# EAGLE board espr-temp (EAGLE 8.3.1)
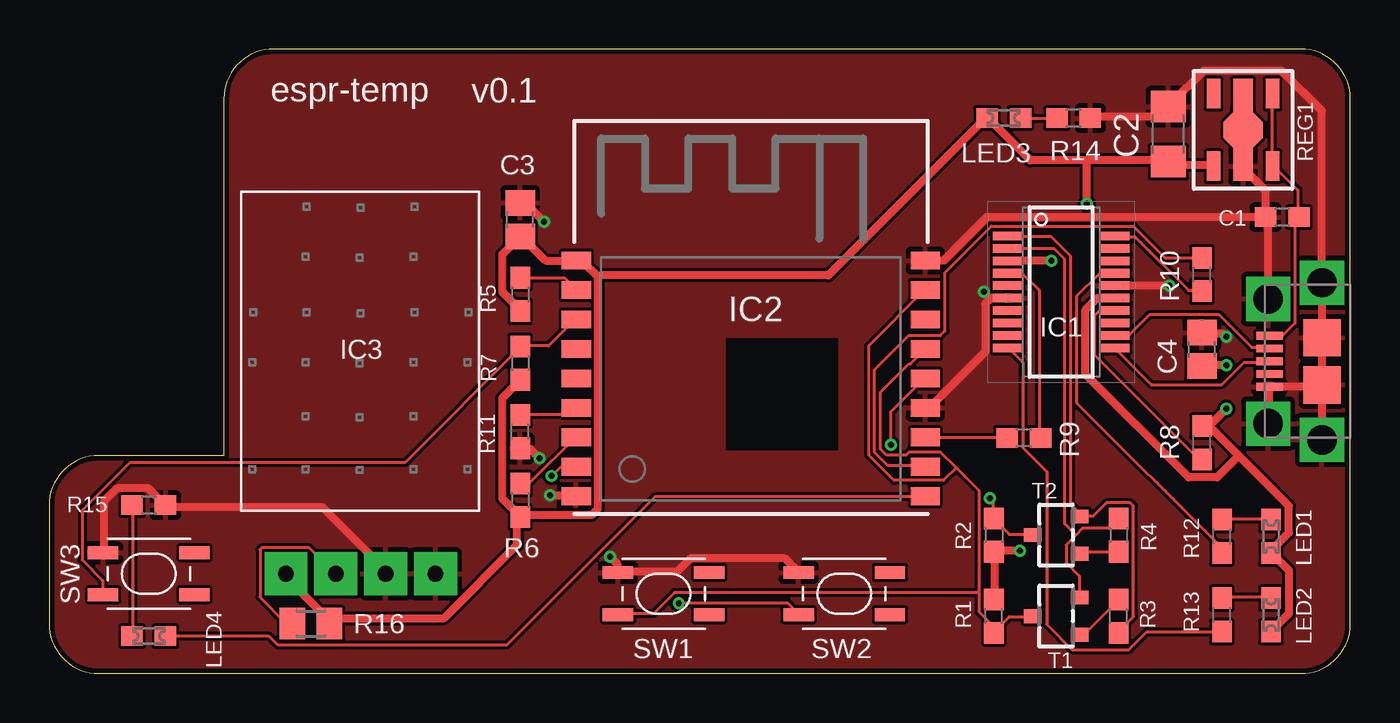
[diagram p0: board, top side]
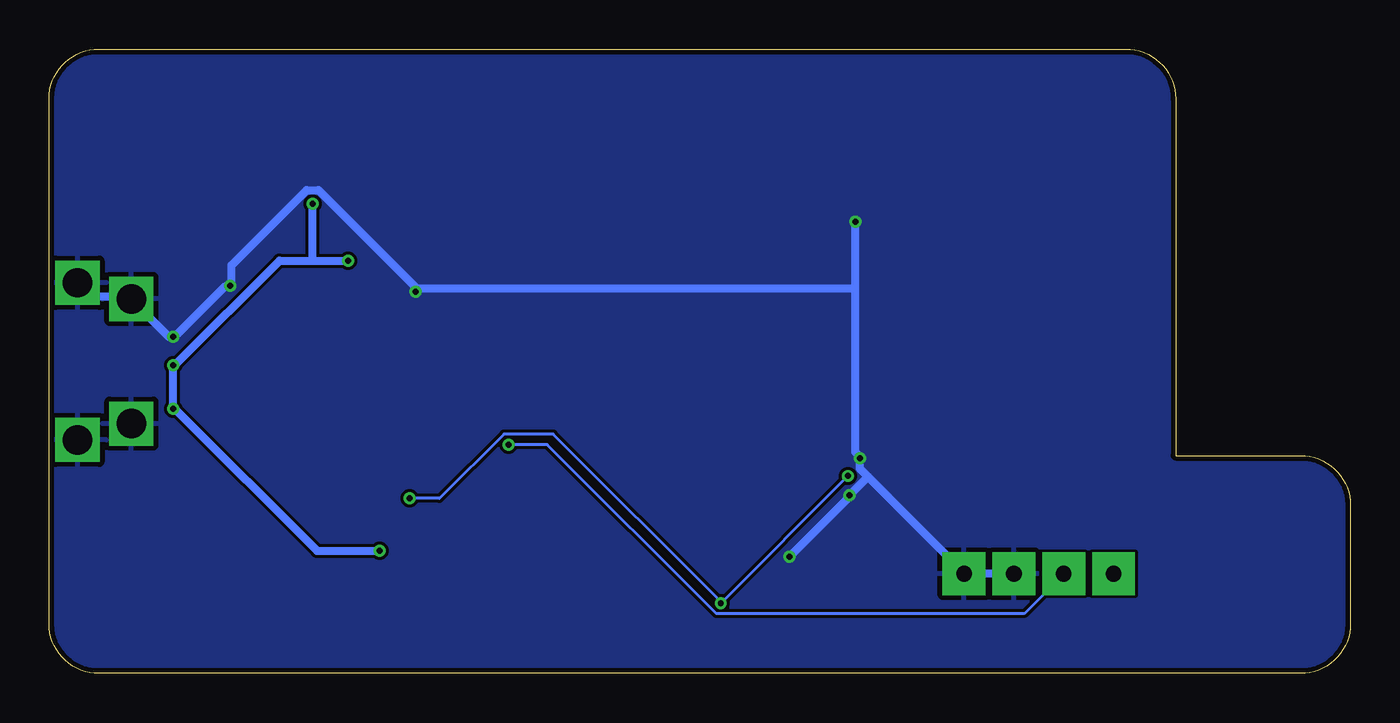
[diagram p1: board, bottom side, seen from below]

Size 66.3 x 31.8 mm. Coordinates in mm from the lower left corner, seen from the top.
Outline: 8.9,11.1 2.54,11.1 arc90 0,8.56 0,2.54 arc90 2.54,0 63.76,0 arc90 66.3,2.54 66.3,29.26 arc90 63.76,31.8 11.44,31.8 arc90 8.9,29.26 8.9,11.1
Copper layers (1*16): Top 0.035mm / dielectric 1.5mm / Bottom 0.035mm
Design rules "SeeedStudio_2layer_DRU_no_angle_20140221": minimum track width 6mil, minimum drill 12mil, track to track 6mil, track to pad 6mil, pad to pad 6mil, via to via 6mil, smd to smd 0mil, copper to edge 10mil, drill to drill 10mil, minimum pad ring 10mil, minimum via ring 6mil, stop-mask expansion 2mil, vias tented up to drill 100mil, thermal gap 10mil
Net classes: 1 GND: width 0.406 mm, drill 0.102 mm, clearance 0.127 mm; 2 3V3: width 0.406 mm, drill 0.102 mm, clearance 0.127 mm

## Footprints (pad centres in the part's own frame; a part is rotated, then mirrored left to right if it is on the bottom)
C1608 = smd 1.1 x 1: 1 -0.85,0; 2 0.85,0
C3216 = smd 1.6 x 1.8: 1 -1.4,0; 2 1.4,0
C2012 = smd 1.3 x 1.5: 1 -0.85,0; 2 0.85,0
SOP64P599X175-20N = smd 1.526 x 0.435: 1 -2.712,2.858; 2 -2.712,2.222; 3 -2.712,1.588; 4 -2.712,0.952; 5 -2.712,0.318; 6 -2.712,-0.318; 7 -2.712,-0.952; 8 -2.712,-1.588; 9 -2.712,-2.222; 10 -2.712,-2.858; 11 2.712,-2.858; 12 2.712,-2.222; 13 2.712,-1.588; 14 2.712,-0.952; 15 2.712,-0.318; 16 2.712,0.318; 17 2.712,0.952; 18 2.712,1.588; 19 2.712,2.222; 20 2.712,2.858
FRONT-FACE = smd 1.485 x 0.9: 1 -8.893,4.9; 2 -8.893,3.4; 3 -8.893,1.9; 4 -8.893,0.4; 5 -8.893,-1.1; 6 -8.893,-2.6; 7 -8.893,-4.1; 8 -8.893,-5.6; 9 -8.893,-7.1; 10 8.893,-7.1; 11 8.893,-5.6; 12 8.893,-4.1; 13 8.893,-2.6; 14 8.893,-1.1; 15 8.893,0.4; 16 8.893,1.9; 17 8.893,3.4; 18 8.893,4.9
AM2320 = drill 0.8 pad 2.184 square: GND 1.27,-11.43; SCL 3.81,-11.43; SDA -1.27,-11.43; VDD -3.81,-11.43
C1608' = smd 1.1 x 1: A 0.85,0; C -0.85,0
R1608 = smd 1.1 x 1: 1 -0.85,0; 2 0.85,0
M0805 = smd 1.3 x 1.6: 1 -0.95,0; 2 0.95,0
SOT-89-5 = smd 0.7 x 1.5: 1 -1.5,-1.85; 3 1.5,-1.85; 4 1.5,1.85; 5 -1.5,1.85 | smd 1 x 1.5: 2 0,-1.85; 2_1 0,1.85 | smd 0.8 x 0.8: 2_0 0,0; 2_4 -0.6,0; 2_5 0.6,0 | smd 1 x 0.5: 2_2 0,0.9; 2_7 0,-0.9 | smd 1.41 x 1.41 rotated 45: 2_3 0,0.4; 2_6 0,-0.4
SKRPACE010 = smd 1.55 x 0.65: 1 -2.325,1.075; 2 2.325,1.075; 3 -2.325,-1.075; 4 2.325,-1.075
SOT346 = smd 0.7 x 0.9: 1 -0.95,-1.2; 2 0.95,-1.2; 3 0,1.2
ZX62B5PA = smd 0.4 x 1.35: D+ 0,4.125; D- 0.65,4.125; GND -1.3,4.125; ID -0.65,4.125; VBUS 1.3,4.125 | drill 1.499 pad 2.032 square: SLD1 -3.175,4.191; SLD2 3.175,4.191; SLD3 -4,1.45; SLD6 4,1.45 | smd 1.9 x 1.9: SLD4 -1.2,1.45; SLD5 1.2,1.45

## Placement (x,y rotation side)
C1  0.39u  [C1608]  62.83,23.24 180 top
C2  4.7u  [C3216]  57.02,27.47 90 top
C3  0.1u  [C2012]  24,23.11 90 top
C4  0.1u  [C2012]  58.74,16.51 90 top
IC1  FT231XS-R  [SOP64P599X175-20N]  51.56,19.43 0 top
IC2  ESP-WROOM-02  [FRONT-FACE]  35.75,16.13 0 top
IC3  AM2320  [AM2320]  15.88,16.51 0 top
LED1  [C1608']  62.26,6.99 270 top
LED2  [C1608']  62.26,2.98 270 top
LED3  [C1608']  48.64,28.3 180 top
LED4  [C1608']  5.08,1.91 0 top
R1  10k  [R1608]  48.13,2.92 90 top
R2  10k  [R1608]  48.13,7.05 270 top
R3  10k  [R1608]  54.48,2.92 90 top
R4  10k  [R1608]  54.48,7.05 270 top
R5  10k  [R1608]  24,19.3 270 top
R6  10k  [R1608]  24,8.83 270 top
R7  10k  [R1608]  24,15.81 270 top
R8  10k  [R1608]  58.74,11.75 90 top
R9  470  [R1608]  49.66,12 180 top
R10  470  [R1608]  58.74,20.32 90 top
R11  10k  [R1608]  24,12.32 90 top
R12  1k  [R1608]  59.75,6.99 90 top
R13  1k  [R1608]  59.75,2.98 90 top
R14  10k  [R1608]  52.2,28.28 180 top
R15  1k  [R1608]  5.08,8.57 180 top
R16  4.7k  [M0805]  13.34,2.54 180 top
REG1  NJM2884U1  [SOT-89-5]  60.83,27.69 180 top
SW1  [SKRPACE010]  31.31,4.06 0 top
SW2  [SKRPACE010]  40.51,4.06 0 top
SW3  [SKRPACE010]  5.08,5.08 0 top
T1  [SOT346]  51.31,2.92 90 top
T2  [SOT346]  51.31,7.05 90 top
USB1  MICRO-USB  [ZX62B5PA]  66.3,15.9 90 top

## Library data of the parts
C1-C4 R16 = rcl
IC1 = FT231XS-R; DESCRIPTION: FTDI Chip FT231XS-R, Interface RS232, RS422, RS485, SIE, UART 3MBd, 5 V, 20-pin, SSOP; HEIGHT: 1.7526mm; MANUFACTURER_NAME: FTDI Chip; MANUFACTURER_PART_NUMBER: FT231XS-R; RS_PART_NUMBER: 7570032P
IC2 = esp-wroom-02
IC3 = am2320
LED1-LED4 = led-smd
R1-R15 = registors
REG1 = regulator
SW1-SW3 = switches
T1 T2 = transistors
USB1 = usb-connector

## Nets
+3V3 [3V3]: C2.1 C3.1 C4.1 IC1.3 IC1.15 IC2.1 IC3.VDD LED1.A LED2.A LED3.A R1.2 R2.2 R5.2 R6.2 R7.2 R8.2 R16.1 REG1.4
CBUS1: IC1.17 R12.1
CBUS2: IC1.10 R13.1
D+: IC1.11 USB1.D+
D-: IC1.12 USB1.D-
DTR: IC1.1 R3.1 T2.2
GND [GND]: C1.2 C2.2 C3.2 C4.2 IC1.6 IC1.16 IC2.9 IC2.13 IC2.18 IC3.GND IC3.SCL R11.1 R14.1 R15.1 REG1.2_1 SW1.1 SW2.1 SW3.1 USB1.GND USB1.SLD1 USB1.SLD2 USB1.SLD3 USB1.SLD4 USB1.SLD5 USB1.SLD6
IO0: IC2.8 R2.1 SW2.3 T2.3
IO4: IC2.10 LED4.A
IO5: IC2.14 IC3.SDA R16.2
N$1: IC2.2 R5.1
N$2: LED4.C R15.2
N$3: IC2.7 R6.1
N$4: C1.1 REG1.1 REG1.5 USB1.VBUS
N$5: LED1.C R12.2
N$6: R3.2 T1.1
N$7: R4.2 T2.1
N$8: LED2.C R13.2
N$9: LED3.C R14.2
N$10: IC2.12 R9.2
N$11: IC2.11 R10.2
N$12: IC2.6 R11.2
N$14: IC1.14 R8.1
N$16: IC2.3 R7.1 SW3.3
RESET: IC2.15 IC2.17 R1.1 SW1.3 T1.3
RTS: IC1.2 R4.1 T1.2
RXD: IC1.4 R9.1
TXD: IC1.20 R10.1

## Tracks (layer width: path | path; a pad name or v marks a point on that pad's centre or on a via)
+3V3  (via drill 0.3)
  Top 0.406: R5.2 24,18.52 23.09,19.43 23.09,21.34 C3.1 24.16,22.17 25.3,21.03 26.82,21.03 IC2.1 27.05,20.95 27.2,20.95 27.96,20.19 | R6.2 24,8 23.09,8.91 23.09,14.02 24,14.94 R7.2 | IC3.VDD 12.12,5.03 12.12,4.88 14.25,2.74 14.25,2.59 R16.1 14.4,2.82 20.12,2.82 23.85,6.55 23.85,7.85 R6.2 | 27.96,20.19 27.96,8.38 27.66,8.08 24.16,8.08 R6.2 | 52.88,26.14 57,26.14 C2.1 57.15,25.91 59.28,25.91 REG1.4 | 52.88,26.14 49.99,26.14 47.85,28.27 LED3.A 47.62,28.19 39.7,20.27 28.12,20.27 27.96,20.19 | R1.2 48.16,3.81 48.16,6.17 R2.2 48.31,6.25 v49.45,6.25 | LED2.A 62.33,2.21 63.17,3.05 63.17,5.26 62.33,6.1 LED1.A 62.33,6.33 63.17,7.16 63.17,8.53 60.62,11.09 | 60.62,11.09 59.13,12.57 58.75,12.57 R8.2 59.21,12.72 v59.97,13.49 | v59.97,15.7 58.75,15.7 C4.1 | v51.05,21.03 48.92,21.03 IC1.3 | 60.62,11.09 59.51,9.98 58.06,9.98 52.81,15.24 52.81,18.52 53.42,19.13 54.25,19.13 IC1.15 | v52.88,23.93 52.88,26.14
  Bottom 0.406: 52.88,21.03 54.56,21.03 59.82,15.77 v59.97,15.7 v59.97,13.49 59.82,13.41 52.65,6.25 v49.45,6.25 | 52.88,21.03 v51.05,21.03 | 52.88,21.03 v52.88,23.93
CBUS1
  Top 0.152: R12.1 59.74,6.17 59.74,6.4 52.35,13.79 52.35,19.2 53.49,20.34 54.25,20.34 IC1.17
CBUS2
  Top 0.152: R13.1 55.93,2.13 55.02,1.22 52.12,1.22 50.83,2.52 50.83,10.29 49.61,11.51 49.61,15.85 48.92,16.54 IC1.10
D+
  Top 0.152: USB1.D+ 62.1,15.85 60.88,15.85 59.74,14.71 56.16,14.71 54.33,16.54 IC1.11
D-
  Top 0.152: USB1.D- 62.1,16.61 61.27,16.61 59.59,18.29 56.08,18.29 55.02,17.22 54.33,17.22 IC1.12
DTR
  Top 0.152: R3.1 54.48,2.13 55.24,2.9 55.24,8.53 55.09,8.69 53.87,8.69 53.19,8 52.58,8 T2.2 52.58,8.08 52.05,8.61 52.05,21.26 51.05,22.25 48.92,22.25 IC1.1
GND  (via drill 0.3)
  Top 0.406: C1.2 61.95,23.24 61.95,24.61 60.88,25.68 60.88,25.83 REG1.2_1 | C1.2 47.78,23.24 45.57,21.03 44.65,21.03 IC2.18 | 47.97,19.09 48.01,19.13 48.84,19.13 IC1.6 | 47.97,19.09 47.7,18.82 47.7,16.38 44.88,13.56 44.65,13.56 IC2.13 | v59.97,17.14 59.82,17.3 58.75,17.3 C4.2 | v57.07,19.74 54.33,19.74 IC1.16 | v47.62,19.43 47.97,19.09 | C1.2 62.1,23.09 62.1,19.13 USB1.SLD2 | USB1.SLD4 64.85,17.07 USB1.SLD5 64.85,17.3 64.85,19.74 USB1.SLD6 64.85,19.96 64.85,28.65 62.79,30.71 58.83,30.71 57.15,29.03 C2.2 57,28.8 56.54,28.35 53.11,28.35 R14.1 | USB1.SLD1 62.18,12.72 62.18,14.55 USB1.GND 62.33,14.63 64.69,14.63 USB1.SLD4 | USB1.SLD3 64.85,11.96 64.85,14.48 USB1.SLD4 | SW3.1 2.82,6.17 2.82,8.76 3.5,9.45 5.03,9.45 5.87,8.61 R15.1 6.1,8.46 13.95,8.46 17.14,5.26 IC3.GND | SW2.1 38.18,5.18 37.49,5.87 32.69,5.87 32,5.18 29.03,5.18 SW1.1 28.96,5.33 28.96,5.56 v28.57,5.94 | v24.99,10.97 24.54,11.43 24,11.43 R11.1 | v25.53,9.07 26.82,9.07 IC2.9 | v25.22,23.01 24.31,23.93 24,23.93 C3.2
  Bottom 0.406: USB1.SLD6 64.85,19.89 64.16,19.2 62.26,19.2 USB1.SLD2 62.1,19.05 60.2,17.14 v59.97,17.14 59.82,17.22 57.3,19.74 v57.07,19.74 57,19.89 57,20.8 53.19,24.61 52.58,24.61 47.62,19.66 v47.62,19.43 47.47,19.58 25.22,19.58 | 24.57,10.02 19.66,5.11 IC3.SCL 19.51,5.11 17.14,5.11 IC3.GND | 24.57,10.02 24.99,10.44 v24.99,10.97 25.07,11.12 25.22,11.28 25.22,19.58 | 24.57,10.02 v25.53,9.07 25.6,8.91 v28.57,5.94 | 25.22,19.58 v25.22,23.01
  pour Top: 67.94,33.02 67.94,-1.27 -1.27,-1.27 -1.27,-0.64 -1.27,33.02
  pour Bottom: 67.31,33.02 67.31,-1.27 -0.64,-1.27 -0.64,-0.64 -0.64,33.02
IO0  (via drill 0.3)
  Top 0.152: T2.3 50.06,7.09 48.92,7.09 48.16,7.85 R2.1 48.08,7.92 48.08,8.76 v47.93,8.91 | v25.6,10.06 26.06,10.52 26.82,10.52 IC2.8 | v32.08,3.58 37.64,3.58 38.18,3.05 SW2.3
  Bottom 0.152: v25.6,10.06 v32.08,3.58 32.08,3.66 40.62,12.19 43.13,12.19 46.41,8.91 v47.93,8.91
IO4
  Top 0.152: LED4.A 11.2,1.91 11.66,1.45 23.32,1.45 30.86,8.99 44.58,8.99 IC2.10
IO5  (via drill 0.3)
  Top 0.152: v42.9,11.66 42.9,13.34 44.58,15.01 IC2.14 | R16.2 12.34,2.59 12.04,2.59 10.74,3.89 10.74,6.33 10.82,6.4 13.26,6.4 14.55,5.11 IC3.SDA
  Bottom 0.152: v42.9,11.66 40.92,11.66 32.31,3.05 16.61,3.05 14.63,5.03 IC3.SDA
N$1
  Top 0.152: R5.1 24,20.12 26.29,20.12 26.82,19.58 IC2.2
N$2
  Top 0.152: LED4.C 4.27,1.91 4.27,8.53 R15.2
N$3
  Top 0.152: R6.1 24.46,9.68 26.82,12.04 IC2.7 | R6.1
N$4
  Top 0.152: 63.63,23.24 63.63,24.61 62.41,25.83 REG1.5 62.33,25.91 62.33,29.49 REG1.1 | 63.63,23.24 63.48,23.09 63.48,17.83 62.87,17.22 62.18,17.22 USB1.VBUS | 63.63,23.24 C1.1
N$5
  Top 0.152: R12.2 59.82,7.85 62.26,7.85 LED1.C
N$6
  Top 0.152: T1.1 52.58,1.98 52.73,1.98 54.48,3.73 R3.2
N$7
  Top 0.152: T2.1 52.58,6.17 54.48,6.17 R4.2
N$8
  Top 0.152: R13.2 59.82,3.89 62.26,3.89 LED2.C
N$9
  Top 0.152: R14.2 51.28,28.27 49.53,28.27 LED3.C
N$10
  Top 0.152: R9.2 48.77,12.04 44.65,12.04 IC2.12
N$11
  Top 0.152: R10.2 58.67,21.18 56.84,21.18 55.24,22.78 48.01,22.78 45.64,20.42 45.64,17.45 45.41,17.22 43.81,17.22 42.06,15.47 42.06,11.28 42.75,10.59 44.58,10.59 IC2.11
N$12
  Top 0.152: R11.2 24,13.18 26.52,13.18 26.82,13.49 IC2.6
N$14
  Top 0.152: R8.1 58.67,10.97 58.52,10.97 53.26,16.23 53.26,18.21 53.49,18.44 54.25,18.44 IC1.14
N$16
  Top 0.152: IC2.3 26.82,18.06 25.45,16.69 24,16.69 R7.1 24,16.61 18.14,10.74 4.12,10.74 1.68,8.31 1.68,5.79 2.74,4.72 2.74,4.04 SW3.3
RESET
  Top 0.152: T1.3 50.06,2.9 48.92,2.9 48.16,2.13 R1.1 48.23,2.29 47.4,3.12 47.4,4.12 | 46.22,10.48 47.4,9.3 47.4,4.12 | 46.22,10.48 45.41,11.28 43.81,11.28 43.66,11.12 42.67,11.12 42.37,11.43 42.37,14.33 43.81,15.77 43.89,15.77 44.58,16.46 IC2.15 | 46.22,10.48 45.57,9.83 43.05,9.83 41.76,11.12 41.76,16.69 44.58,19.51 IC2.17 | 47.4,4.12 31.85,4.12 30.79,3.05 29.03,3.05 SW1.3
RTS
  Top 0.152: 52.31,7.05 52.65,7.39 54.03,7.39 54.48,7.85 R4.1 | 52.31,7.05 51.82,6.55 51.82,5.64 52.5,4.95 52.5,3.89 T1.2 | 52.31,7.05 51.74,7.62 51.74,21.11 51.21,21.64 48.92,21.64 IC1.2
RXD
  Top 0.152: R9.1 50.44,12.04 50.44,19.51 49.61,20.34 48.92,20.34 IC1.4
TXD
  Top 0.152: R10.1 58.67,19.51 58.06,19.51 55.32,22.25 54.33,22.25 IC1.20

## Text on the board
tPlace: espr-temp | v0.1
